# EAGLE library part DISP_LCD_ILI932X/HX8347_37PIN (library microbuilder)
37-pin 2.8" 240x320 Displays based on ILI9325/ILI9328/HX8347 Controllers Make sure to double-check the footprint against any LCD since there are dozens of varieties, but this footprint uses a relatively common 37-pin layout for ILI9325, ILI9328 or HX9347 240x320 LCD displays.
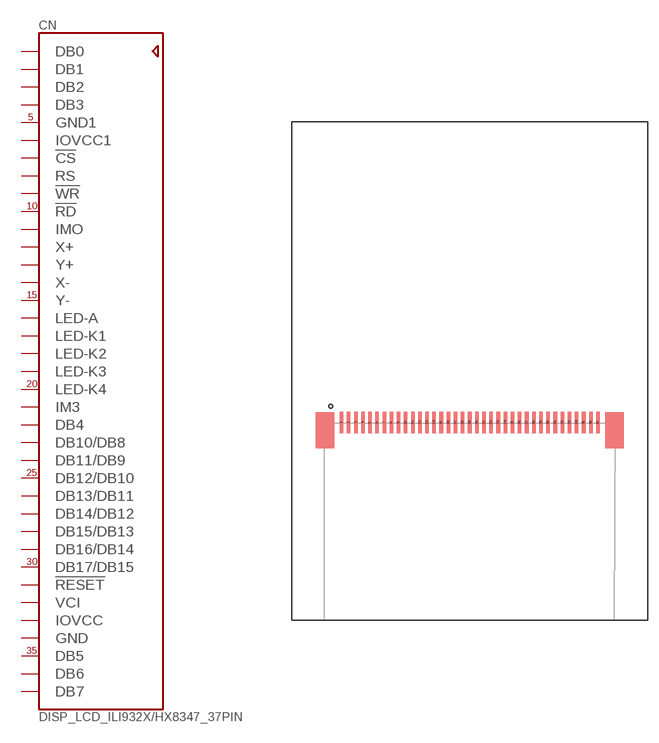
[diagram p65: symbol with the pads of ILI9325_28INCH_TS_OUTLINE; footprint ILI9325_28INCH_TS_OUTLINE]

Designator prefix CN

## DISP_LCD_ILI932X/HX8347_37PINOUTLINE  [ILI9325_28INCH_TS_OUTLINE]
1  DB0  pas
2  DB1  pas
3  DB2  pas
4  DB3  pas
5  GND1  pwr
6  IOVCC1  pwr
7  !CS  pas
8  RS  pas
9  !WR  pas
10  !RD  pas
11  IMO  pas
12  X+  pas
13  Y+  pas
14  X-  pas
15  Y-  pas
16  LED-A  pas
17  LED-K1  pas
18  LED-K2  pas
19  LED-K3  pas
20  LED-K4  pas
21  IM3  pas
22  DB4  pas
23  DB10/DB8  pas
24  DB11/DB9  pas
25  DB12/DB10  pas
26  DB13/DB11  pas
27  DB14/DB12  pas
28  DB15/DB13  pas
29  DB16/DB14  pas
30  DB17/DB15  pas
31  !RESET  pas
32  VCI  pwr
33  IOVCC  pwr
34  GND  pwr
35  DB5  pas
36  DB6  pas
37  DB7  pas

## Footprint ILI9325_28INCH_TS_OUTLINE (pad centres in mm)
smd 0.5 x 3: 1 -18,27.77; 2 -17,27.77; 3 -16,27.77; 4 -15,27.77; 5 -14,27.77; 6 -13,27.77; 7 -12,27.77; 8 -11,27.77; 9 -10,27.77; 10 -9,27.77; 11 -8,27.77; 12 -7,27.77; 13 -6,27.77; 14 -5,27.77; 15 -4,27.77; 16 -3,27.77; 17 -2,27.77; 18 -1,27.77; 19 0,27.77; 20 1,27.77; 21 2,27.77; 22 3,27.77; 23 4,27.77; 24 5,27.77; 25 6,27.77; 26 7,27.77; 27 8,27.77; 28 9,27.77; 29 10,27.77; 30 11,27.77; 31 12,27.77; 32 13,27.77; 33 14,27.77; 34 15,27.77; 35 16,27.77; 36 17,27.77; 37 18,27.77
